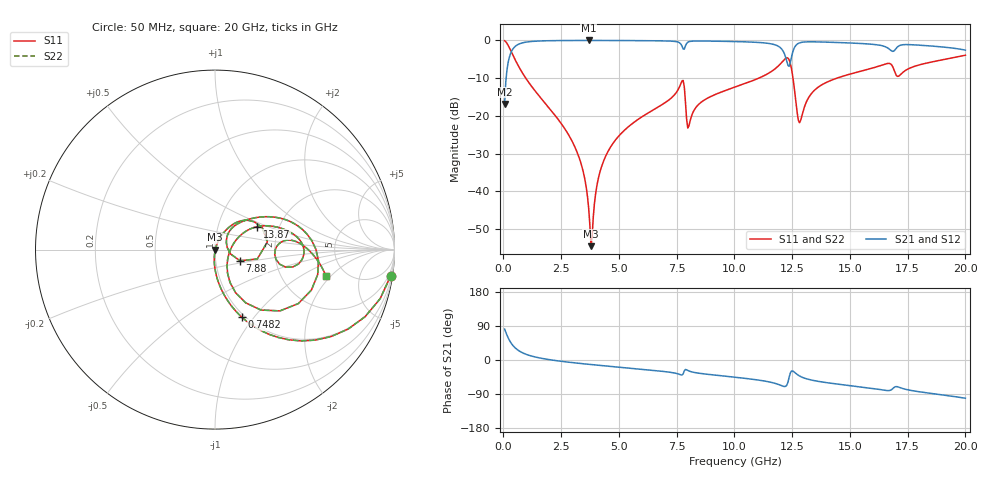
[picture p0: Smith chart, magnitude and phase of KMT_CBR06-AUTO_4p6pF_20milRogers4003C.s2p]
! Data measured by Modelithics Inc. support@modelithics.com 813-866-6335
! KEMET CBR06-AUTO 4.6pF, Pad Width= 0.851mm, Pad Length= 0.64mm, Pad Gap= 0.62mm, 20mil Rogers 4003C substrate Data, January 2022
# hz S ma R 50
! 2 Port Network Data from SP1.SP block
! freq  magS11  angS11  magS21  angS21  magS12  angS12  magS22  angS22
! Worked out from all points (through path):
!   401 points, 50 MHz to 20 GHz, reference 50 ohm
!   highest |S21| = -0.02 dB at 3.691 GHz (marker M1); lowest = -16.8 dB at 50 MHz (marker M2)
!   group delay of S21, straight-line fit = 15.6 ps
!   lowest |S11| = -54.5 dB at 3.791 GHz (marker M3), VSWR 1.00, Z = 50.2 - j0.0995 ohm
!   |S11| at or under -10 dB: 965.4 MHz to 11.06 GHz (10.09 GHz wide, 168 % of centre); 12.53 GHz to 14.44 GHz (1.905 GHz wide, 14.1 % of centre)
!   |S22| runs from -54.5 to -0.1 dB; largest |S21 - S12| = 0
!   S11 on the Smith chart (normalised r, x): 50 MHz: 1, -13; 748.2 MHz: 0.97, -0.87; 7.88 GHz: 1.31, -0.17; 13.87 GHz: 1.54, +0.42; 20 GHz: 3.55, -1.77
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5e7  0.9895 -8.4  0.1441 81.5  0.1441 81.5  0.9895 -8.4
2.99375e8  0.7513 -42.2  0.6591 47.8  0.6591 47.8  0.7513 -42.2
7.4825e8  0.4038 -68.4  0.9139 21.4  0.9139 21.4  0.4038 -68.4
3.391625e9  0.02152 -95.1  0.998 -9.5  0.998 -9.5  0.02152 -95.1
3.690875e9  0.005918 -84.3  0.9981 -11.4  0.9981 -11.4  0.005918 -84.3
3.790625e9  0.001875 -31.9  0.9981 -12.0  0.9981 -12.0  0.001875 -31.9
4.13975e9  0.01626 69.4  0.9979 -14.1  0.9979 -14.1  0.01626 69.4
4.588625e9  0.0365 70.3  0.9972 -16.6  0.9972 -16.6  0.0365 70.3
6.73325e9  0.133 59.6  0.9874 -28.9  0.9874 -28.9  0.133 59.6
7.73075e9  0.2905 25.2  0.8412 -39.7  0.8412 -39.7  0.2905 25.2
7.880375e9  0.1523 -24.0  0.8475 -25.0  0.8475 -25.0  0.1523 -24.0
8.03e9  0.07373 30.7  0.9605 -29.0  0.9605 -29.0  0.07373 30.7
1.0025e10  0.2407 43.4  0.9652 -45.4  0.9652 -45.4  0.2407 43.4
1.18205e10  0.4354 21.9  0.86 -62.7  0.86 -62.7  0.4354 21.9
1.226938e10  0.5888 -13.7  0.5254 -66.2  0.5254 -66.2  0.5888 -13.7
1.246888e10  0.4235 -52.7  0.5966 -29.3  0.5966 -29.3  0.4235 -52.7
1.2818e10  0.08105 -15.3  0.9265 -42.1  0.9265 -42.1  0.08105 -15.3
1.336662e10  0.203 30.7  0.958 -53.3  0.958 -53.3  0.203 30.7
1.386538e10  0.2663 28.6  0.9508 -58.6  0.9508 -58.6  0.2663 28.6
1.670825e10  0.4952 -3.4  0.7652 -80.6  0.7652 -80.6  0.4952 -3.4
1.710725e10  0.3358 -0.1  0.8404 -71.5  0.8404 -71.5  0.3358 -0.1
2e10  0.6361 -13.5  0.7427 -100.9  0.7427 -100.9  0.6361 -13.5
